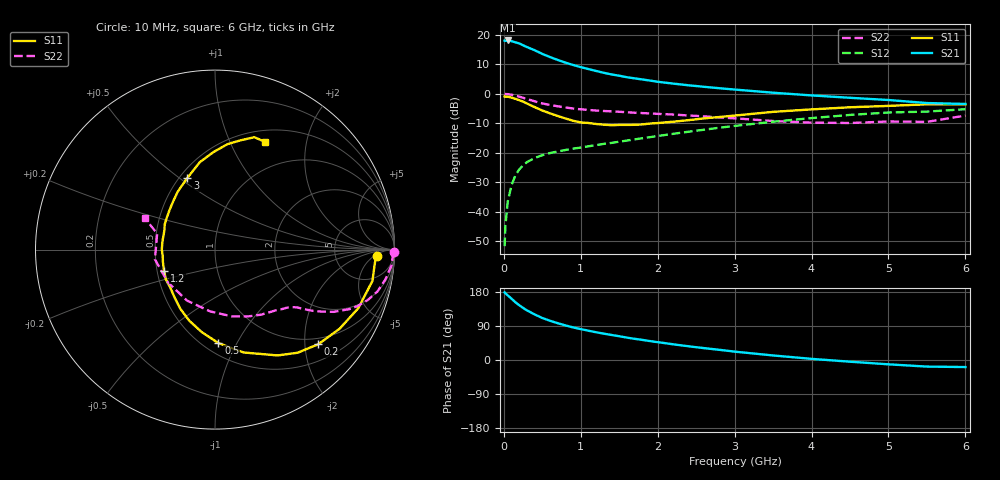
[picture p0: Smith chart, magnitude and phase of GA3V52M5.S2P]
! Infineon Technologies  Discrete & RF Semiconductors
! BF775
! Si NPN RF Bipolar Junction Transistor in SOT23
! VCE = 3.5 V  IC = 2.5 mA
! Common Emitter S-Parameters:  May  1996
# GHz  S  MA  R  50
!  f  S11  S21  S12  S22
! GHz  MAG  ANG  MAG  ANG  MAG  ANG  MAG  ANG
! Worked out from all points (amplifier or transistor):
!   36 points, 10 MHz to 6 GHz, reference 50 ohm
!   highest |S21| = 18.1 dB at 50 MHz (marker M1)
!   |S21| within 3 dB of that: start of sweep to 371.2 MHz
!   unconditionally stable (mu >= 1): 1.077 GHz to 3.601 GHz
!   at 250 MHz: K = 0.33, MSG = 20.4 dB, |S12| = -24.3 dB
!   at 1.4 GHz: K = 1.12, MAG = 9.5 dB, |S12| = -16.7 dB
!   at 6 GHz: K = 0.98, MSG = 0.9 dB, |S12| = -5.2 dB
!   S11 on the Smith chart (normalised r, x): 10 MHz: 17, -6; 200 MHz: 0.85, -2.30; 500 MHz: 0.59, -0.84; 1.2 GHz: 0.54, -0.14; 3 GHz: 0.55, +0.53; 6 GHz: 0.64, +1.36
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0.01  0.9011 -2.3  7.984 178.3  0.0026 89.5  0.9966 -0.9
0.02  0.8943 -4.4  7.89 176.1  0.0057 86.5  0.9912 -2.0
0.05  0.8942 -11.3  8.039 170.7  0.0146 83.2  0.9874 -5.1
0.1  0.8623 -22.3  7.824 161.8  0.0283 78.5  0.9635 -10.0
0.15  0.8225 -32.4  7.474 152.4  0.0413 71.8  0.9352 -14.4
0.2  0.7805 -42.5  7.163 144.6  0.0521 67.1  0.896 -18.3
0.25  0.7363 -51.3  6.663 137.4  0.0612 62.4  0.8558 -21.5
0.3  0.6851 -59.4  6.218 131.0  0.0693 59.5  0.8188 -23.9
0.4  0.5947 -74.5  5.491 120.3  0.0815 54.5  0.7463 -27.7
0.5  0.521 -87.9  4.756 110.8  0.0908 51.2  0.6867 -30.2
0.6  0.4663 -99.0  4.198 103.6  0.0988 48.9  0.6463 -31.9
0.8  0.3821 -120.4  3.381 91.3  0.1113 47.2  0.587 -34.1
0.9  0.3493 -130.1  3.085 86.0  0.1174 47.3  0.5632 -35.0
1.1  0.32 -149.1  2.627 77.3  0.1287 47.8  0.5323 -37.2
1.2  0.3073 -157.5  2.44 73.2  0.1347 48.0  0.5204 -38.3
1.6  0.2963 171.9  1.911 59.1  0.1611 48.9  0.487 -43.6
2.2  0.336 138.9  1.491 41.5  0.2092 49.2  0.4451 -54.5
3  0.4272 111.2  1.181 22.1  0.2853 44.8  0.384 -75.7
3.5  0.4942 99.9  1.044 12.0  0.3359 40.1  0.3454 -94.5
4.5  0.5912 83.3  0.856 -4.5  0.4384 27.8  0.3197 -145.4
5.5  0.6636 70.7  0.697 -17.4  0.4995 12.1  0.3344 164.5
6  0.6616 65.3  0.673 -18.6  0.5477 7.7  0.4269 156.0
